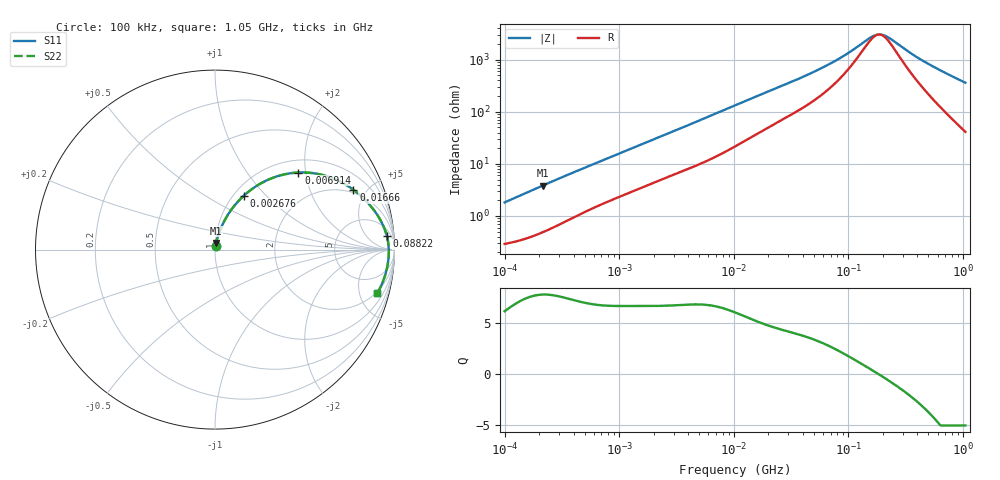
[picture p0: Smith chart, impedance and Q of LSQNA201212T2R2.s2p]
! LSQNA201212T2R2  S-PARAMETER MODEL  ( General Type )
! Model Generated by TAIYO YUDEN Corporation (http://www.ty-top.com)
! Version 2.0
! TAIYO YUDEN Control No. 100810NF25SB-FKC
! Copyright(c) 2007 TAIYO YUDEN CO.,LTD. All Rights Reserved.
! Product Description (link to TY-COMPAS)
! https://ds.yuden.co.jp/TYCOMPAS/or/detail?pn=LSQNA201212T2R2M&u=M
! Products Name : Inductors
! Characteristics :
!  Inductance : 2.2 uH , SRF(min) : 80 MHz , DC Resistance(max) : 0.299 Ohm
!  Rated Current : Saturation :410 mA , Temp Rise : 770 mA (40 degC)
!  Case Size : 2.0 x 1.25 / 0.079 x 0.049 [mm/inch] , Thickness : 1.25 / 0.049 [mm/inch]
!  (Conditions: Temperature = 25 degC , DC Bias Current/Voltage = 0A / 0V)
! External Node Assignments :
!  1  o---GGG---o  2
! GND o---------o GND
! Frequency Range : 0.1MHz  -  1050.104495MHz  [ 402 STEP ]
# MHz S RI R 50
! Freq[MHz].  S11 Real  S11 Imag  S21 Real  S21 Imag  S12 Real  S12 Imag  S22 Real  S22 Imag
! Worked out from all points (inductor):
!   401 points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, 100 kHz to 1.05 GHz, reference 50 ohm
!   read as one part in series: L = 2.85 uH near 104.7 kHz
!   highest Q = 7.82 at 214.7 kHz (marker M1), where L = 2.82 uH
!   self-resonance near 185.1 MHz
!   S11 on the Smith chart (normalised r, x): 100 kHz: 1.01, +0.04; 2.676 MHz: 1.11, +0.76; 6.914 MHz: 1.27, +1.82; 16.66 MHz: 1.80, +4.08; 88.22 MHz: 11, +21; 1.05 GHz: 1.82, -7.18
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0.1  0.00322 0.0179  0.9968 -0.0179  0.9968 -0.0179  0.00322 0.0179
0.21466  0.00625 0.0376  0.9937 -0.0376  0.9937 -0.0376  0.00625 0.0376
0.471581  0.0171 0.077  0.9829 -0.077  0.9829 -0.077  0.0171 0.077
1.163126  0.0545 0.1644  0.9455 -0.1644  0.9455 -0.1644  0.0545 0.1644
2.223888  0.1275 0.2672  0.8725 -0.2672  0.8725 -0.2672  0.1275 0.2672
2.676317  0.1616 0.3013  0.8384 -0.3013  0.8384 -0.3013  0.1616 0.3013
4.154761  0.2755 0.3797  0.7245 -0.3797  0.7245 -0.3797  0.2755 0.3797
6.913753  0.4643 0.4294  0.5357 -0.4294  0.5357 -0.4294  0.4643 0.4294
10.24746  0.6201 0.41  0.3799 -0.41  0.3799 -0.41  0.6201 0.41
16.66215  0.7712 0.3335  0.2288 -0.3335  0.2288 -0.3335  0.7712 0.3335
27.09229  0.866 0.2443  0.134 -0.2443  0.134 -0.2443  0.866 0.2443
48.32509  0.9289 0.1507  0.0711 -0.1507  0.0711 -0.1507  0.9289 0.1507
66.82144  0.9481 0.1067  0.0519 -0.1067  0.0519 -0.1067  0.9481 0.1067
88.21711  0.9582 0.0737  0.0418 -0.0737  0.0418 -0.0737  0.9582 0.0737
150.2359  0.9672 0.0196  0.0328 -0.0196  0.0328 -0.0196  0.9672 0.0196
168.6705  0.9679 0.0087  0.0321 -0.0087  0.0321 -0.0087  0.9679 0.0087
193.8017  0.9684 -0.00427  0.0316 0.00427  0.0316 0.00427  0.9684 -0.00427
227.892  0.9684 -0.0196  0.0316 0.0196  0.0316 0.0196  0.9684 -0.0196
337.7781  0.9656 -0.0597  0.0344 0.0597  0.0344 0.0597  0.9656 -0.0597
456.3747  0.9599 -0.0958  0.0401 0.0958  0.0401 0.0958  0.9599 -0.0958
708.4841  0.9414 -0.1627  0.0586 0.1627  0.0586 0.1627  0.9414 -0.1627
1050.104  0.9052 -0.2412  0.0948 0.2412  0.0948 0.2412  0.9052 -0.2412
